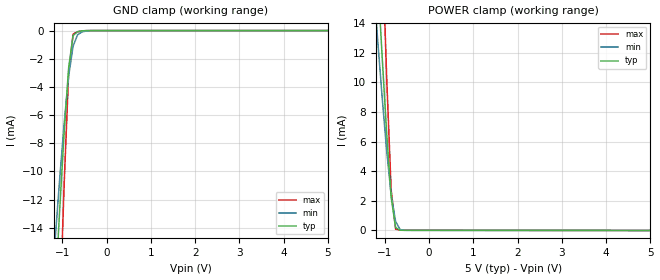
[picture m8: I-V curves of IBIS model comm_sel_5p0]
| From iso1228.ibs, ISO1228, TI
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|   Model comm_sel_5p0
[Model] comm_sel_5p0
Model_type Input
Vinl =  1.500V
Vinh =  3.500V
C_comp   0.525pF   0.628pF   0.413pF
[Model Spec]
Vinh   3.500V   3.150V   3.850V
Vinl   1.500V   1.350V   1.650V
[Temperature Range]   27.000   0.150k   -40.000
[Voltage Range]   5.000V   4.500V   5.500V
[POWER Clamp Reference]   5.000V   4.500V   5.500V
[GND Clamp Reference]   0.0V   0.0V   0.0V
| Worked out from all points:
|   GND clamp passes 1 mA (typ) near -0.79 V on its own axis
|   POWER clamp passes 1 mA (typ) near -0.80 V on its own axis
[GND_clamp]
|Voltage   I(typ)   I(min)   I(max)
-5V       -427.1mA   -303.5mA   -743.3mA
-1.162V   -18.56mA   -14.79mA   -30.25mA
-1.061V   -12.73mA   -10.53mA   -20.31mA
-960mV    -7.235mA   -6.59mA    -10.91mA
-859mV    -2.664mA   -3.241mA   -3.051mA
-758mV    -356.7uA   -1.105mA   -244.4uA
-657mV    -70.53uA   -299.2uA   -89.22uA
-556mV    -18.81uA   -92.55uA   -27.65uA
-354mV    -754.9nA   -4.854uA   -930.9nA
5V        0A         0A         0A
[POWER_clamp]
|Voltage   I(typ)   I(min)   I(max)
-5V       408.8mA    285.1mA    753.8mA
-1.263V   22.71mA    16.85mA    38.69mA
-1.162V   17.13mA    12.83mA    28.94mA
-1.061V   11.7mA     8.972mA    19.42mA
-960mV    6.584mA    5.402mA    10.38mA
-859mV    2.275mA    2.444mA    2.773mA
-758mV    198.2uA    617.9uA    92.31uA
-657mV    17.37uA    63.81uA    17.02uA
-556mV    11.52uA    12.75uA    15.73uA
5V        0A         0A         1.293uA
